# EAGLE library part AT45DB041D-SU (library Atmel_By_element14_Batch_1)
4-megabit DataFlash
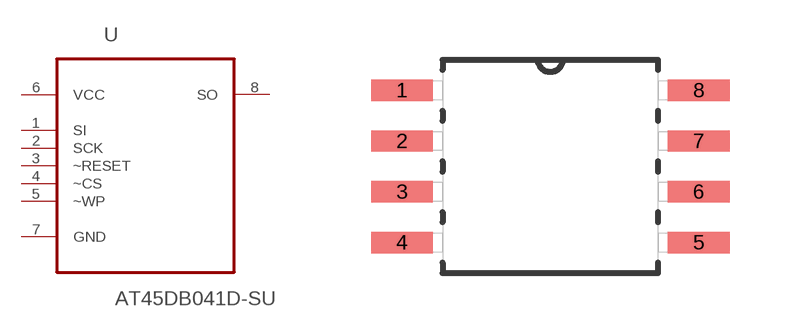
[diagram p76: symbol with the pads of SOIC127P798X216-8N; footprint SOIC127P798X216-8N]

Designator prefix U

## AT45DB041D-SU (MPN: AT45DB041D-SU; OC_FARNELL: 1362661; OC_NEWARK: 50M3333; PACKAGE: SOIC-8; SUPPLIER: Atmel)  [SOIC127P798X216-8N]
1  SI  in
2  SCK  in
3  ~RESET  in
4  ~CS  in
5  ~WP  in
6  VCC  pwr
7  GND  pas
8  SO  out

## Footprint SOIC127P798X216-8N (pad centres in mm)
smd 1.549 x 0.533: 1 -3.708,1.905; 2 -3.708,0.635; 3 -3.708,-0.635; 4 -3.708,-1.905; 5 3.708,-1.905; 6 3.708,-0.635; 7 3.708,0.635; 8 3.708,1.905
